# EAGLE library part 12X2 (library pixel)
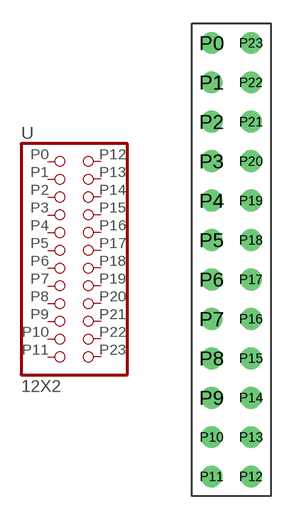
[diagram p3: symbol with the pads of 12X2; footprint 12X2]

Designator prefix -

## 12X2  [12X2]
P0  P0  pas
P1  P1  pas
P2  P2  pas
P3  P3  pas
P4  P4  pas
P5  P5  pas
P6  P6  pas
P7  P7  pas
P8  P8  pas
P9  P9  pas
P10  P10  pas
P11  P11  pas
P12  P12  pas
P13  P13  pas
P14  P14  pas
P15  P15  pas
P16  P16  pas
P17  P17  pas
P18  P18  pas
P19  P19  pas
P20  P20  pas
P21  P21  pas
P22  P22  pas
P23  P23  pas

## Footprint 12X2 (pad centres in mm)
drill 0.9 pad 1.27: P0 -1.27,13.97; P1 -1.27,11.43; P2 -1.27,8.89; P3 -1.27,6.35; P4 -1.27,3.81; P5 -1.27,1.27; P6 -1.27,-1.27; P7 -1.27,-3.81; P8 -1.27,-6.35; P9 -1.27,-8.89; P10 -1.27,-11.43; P11 -1.27,-13.97; P12 1.27,-13.97; P13 1.27,-11.43; P14 1.27,-8.89; P15 1.27,-6.35; P16 1.27,-3.81; P17 1.27,-1.27; P18 1.27,1.27; P19 1.27,3.81; P20 1.27,6.35; P21 1.27,8.89; P22 1.27,11.43; P23 1.27,13.97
